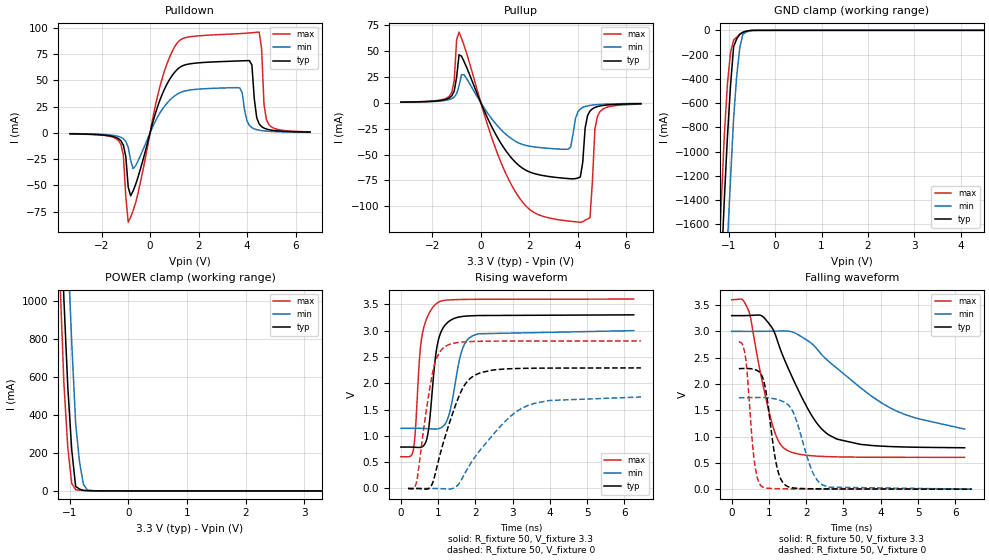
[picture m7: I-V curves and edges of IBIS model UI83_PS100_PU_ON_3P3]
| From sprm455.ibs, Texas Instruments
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|   Model Cell UI83_PS100_PU_ON_3P3
|IDG09_OUI83_PS100_PU_ON_3P3
[Model]   UI83_PS100_PU_ON_3P3
Model_type   I/O
Polarity   Non-Inverting
Enable   Active-Low
Vinl =  0.8V
Vinh =  2V
Cref =  15pF
Rref =  100.00M
Vref =  0V
Vmeas =  1.65
C_comp   5.307p   5.123p   6.171p
[Model Spec]
Vinl   0.8V   0.8V   0.8V
Vinh   2V   2V   2V
[Temperature Range]   25   125   -40
[Voltage Range]   3.3   3   3.6
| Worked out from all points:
|   slope of the pulldown table from 0 to 0.495 V, typ, clamps not added: 13.6 ohm
|   slope of the pullup table from 0 to 0.495 V, typ, clamps not added: 19.6 ohm
|   GND clamp passes 1 mA (typ) near -0.51 V on its own axis
|   POWER clamp passes 1 mA (typ) near -0.67 V on its own axis
|   rising waveform, R_fixture 50, V_fixture 3.3: 20-80 % time 228ps typ, 309ps min, 197ps max; typ from 0.787 V to 3.3 V
|   rising waveform, R_fixture 50, V_fixture 0: 20-80 % time 625ps typ, 1.21ns min, 356ps max; typ from 0 V to 2.29 V
|   falling waveform, R_fixture 50, V_fixture 3.3: 20-80 % time 1.01ns typ, 2.01ns min, 532ps max; typ from 3.3 V to 0.787 V
|   falling waveform, R_fixture 50, V_fixture 0: 20-80 % time 277ps typ, 463ps min, 193ps max; typ from 2.29 V to 0 V
| Nom Voltages:
|   VDD=1.1, VDDS=3.3, VSS=0, VSSS=0
| Min Voltages:
|   VDD=1, VDDS=3, VSS=0, VSSS=0
| Max Voltages:
|   VDD=1.2, VDDS=3.6, VSS=0, VSSS=0
[POWER_clamp]
|   voltage   I(typ)   I(min)   I(max)
-3.3V     22.22A     22.93A     21.83A
-1.167V   1.575A     2.376A     1.114A
-1.1V     1.013A     1.799A     568.4mA
-1.033V   547.6mA    1.267A     227.3mA
-966.7mV  217.9mA    785.9mA    39.8mA
-900mV    23.47mA    356.5mA    5.728mA
-833.3mV  9.703mA    151.6mA    4.044mA
-766.7mV  2.302mA    34.24mA    2.667mA
-700mV    1.264mA    4.305mA    1.595mA
-366.7mV  36.71uA    46.16uA    51.38uA
3.3V      -113.8uA   -88.61uA   -192.6uA
[Pulldown]
|   voltage   I(typ)   I(min)   I(max)
-3.3V     -826.1uA   -650.2uA   -901.2uA
-1.3V     -5.507mA   -3.361mA   -7.401mA
-1.1V     -11.64mA   -5.587mA   -21.31mA
-900mV    -51.57mA   -13.7mA    -84.93mA
-700mV    -55.24mA   -34.01mA   -74.16mA
1.1V      59.92mA    36.57mA    85.06mA
3.7V      68.51mA    42.82mA    94.48mA
4.1V      68.76mA    7.013mA    95.13mA
4.5V      8.571mA    2.593mA    95.94mA
4.7V      4.569mA    1.949mA    26.88mA
4.9V      3.077mA    1.558mA    8.021mA
6.6V      795.1uA    568.4uA    1.029mA
[Pullup]
|   voltage   I(typ)   I(min)   I(max)
-3.3V     663.7uA    556.1uA    740.7uA
-1.3V     4.799mA    3.15mA     6.471mA
-1.1V     11.28mA    5.644mA    21.14mA
-1V       24.69mA    8.858mA    61.1mA
-900mV    46.52mA    16.5mA     68.38mA
1.5V      -59.13mA   -38.08mA   -88.85mA
3.6V      -73.21mA   -44.75mA   -114.2mA
4.1V      -71.75mA   -5.995mA   -115.4mA
4.5V      -7.928mA   -2.493mA   -111mA
4.7V      -4.5mA     -1.913mA   -26.06mA
4.9V      -3.111mA   -1.549mA   -8.885mA
6.6V      -838.9uA   -584.8uA   -1.219mA
[GND_clamp]
|   voltage   I(typ)   I(min)   I(max)
-3.3V     -22.66A    -23.52A    -22.18A
-1.233V   -2.568A    -3.511A    -2.016A
-1.167V   -1.975A    -2.911A    -1.431A
-1.1V     -1.395A    -2.319A    -866.2mA
-1.033V   -879.2mA   -1.758A    -444.8mA
-966.7mV  -459.2mA   -1.228A    -183.4mA
-900mV    -135.2mA   -728.2mA   -82.02mA
-833.3mV  -71.2mA    -377.8mA   -56.78mA
-766.7mV  -31.56mA   -145.7mA   -34.97mA
-700mV    -16.27mA   -32.05mA   -16.57mA
-366.7mV  -134.3uA   -203.6uA   -197.3uA
6.6V      0A         0A         0A
[Ramp]
| variable   typ   min   max
dV/dt_f  1.5141217/1.0134233n  1.1185831/2.0095542n  1.8053632/0.53292308n
dV/dt_r   1.382451/0.6265857n  1.0500356/1.2130705n  1.6901199/0.3570789n
R_load = 50
[Rising Waveform]
R_fixture = 50
V_fixture = 3.3
V_fixture_min = 3
V_fixture_max = 3.6
|   time   V(typ)   V(min)   V(max)
0s        787.2mV    1.143V     605.4mV
334.7ps   785.5mV    1.144V     735.5mV
394.2ps   783.1mV    1.144V     1.151V
518.7ps   781.4mV    1.142V     2.627V
673ps     889mV      1.139V     3.19V
980ps     2.735V     1.133V     3.528V
1.267ns   3.163V     1.344V     3.583V
1.625ns   3.267V     2.592V     3.592V
1.925ns   3.283V     2.902V     3.595V
6.25ns    3.3V       3V         3.6V
[Rising Waveform]
R_fixture = 50
V_fixture = 0
V_fixture_min = 0
V_fixture_max = 0
|   time   V(typ)   V(min)   V(max)
192.1ps   0V         0V         0V
427.2ps   0V         0V         144.5mV
804.7ps   39.7mV     0V         2.024V
980.8ps   447.3mV    0V         2.511V
1.246ns   1.119V     -10.66mV   2.721V
1.702ns   1.957V     267.2mV    2.786V
2.173ns   2.207V     768.7mV    2.798V
2.933ns   2.276V     1.366V     2.802V
3.576ns   2.286V     1.616V     2.803V
6.442ns   2.291V     1.739V     2.804V
[Falling Waveform]
R_fixture = 50
V_fixture = 3.3
V_fixture_min = 3
V_fixture_max = 3.6
|   time   V(typ)   V(min)   V(max)
0s        3.3V       3V         3.6V
278.2ps   3.299V     3V         3.609V
459.9ps   3.302V     3V         3.38V
786.1ps   3.302V     3.001V     2.163V
1.044ns   3.108V     3.003V     1.351V
1.411ns   2.469V     3.007V     774.2mV
2.208ns   1.333V     2.729V     631.8mV
2.827ns   951.1mV    2.297V     613.9mV
4.398ns   806.5mV    1.494V     605.9mV
6.25ns    787.2mV    1.143V     605.4mV
[Falling Waveform]
R_fixture = 50
V_fixture = 0
V_fixture_min = 0
V_fixture_max = 0
|   time   V(typ)   V(min)   V(max)
192.1ps   2.291V     1.739V     2.804V
358.2ps   2.295V     1.739V     2.561V
607.7ps   2.276V     1.743V     537.2mV
821.6ps   2.137V     1.742V     44.88mV
940.3ps   1.769V     1.738V     20.18mV
1.206ns   445.9mV    1.708V     9.483mV
1.506ns   49.13mV    1.609V     6.227mV
2.158ns   7.619mV    346.7mV    3.127mV
2.439ns   5.618mV    80.33mV    2.491mV
6.442ns   0V         0V         0V
